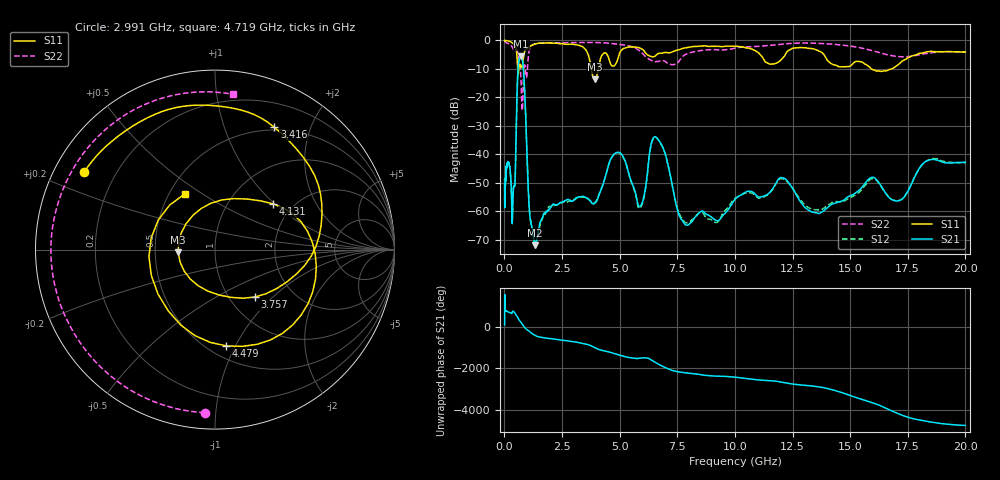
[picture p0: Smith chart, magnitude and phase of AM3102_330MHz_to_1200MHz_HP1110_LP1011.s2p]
! Date/Time: Tue, Sep 11, 2018 5:23 PM
! Network Analyzer: Agilent Technologies E8362B Rev: A.07.50.63
! Sweep from 0.010 to 20.000 GHz, 1601 Points, Sweep Type: LOG
! Power Supply: 4.949 V, 0.001 A
# Hz S DB R 50
!freq MagS11 AngS11 MagS21 AngS21 MagS12 AngS12 MagS22 AngS22
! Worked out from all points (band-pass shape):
!   1601 points, 10 MHz to 20 GHz, reference 50 ohm
!   highest |S21| = -5.65 dB at 726 MHz (marker M1); lowest = -72.0 dB at 1.34 GHz (marker M2)
!   |S21| within 3 dB of the highest: 603.5 MHz to 810.2 MHz (206.7 MHz wide, 29.2 % of centre)
!   lowest |S11| = -13.7 dB at 3.921 GHz (marker M3), VSWR 1.52, Z = 33 - j1.1 ohm
!   |S11| at or under -10 dB: 573.5 MHz to 626 MHz (52.43 MHz wide, 8.74 % of centre); 3.772 GHz to 4.081 GHz (308.9 MHz wide, 7.87 % of centre); 15.91 GHz to 16.81 GHz (895.3 MHz wide, 5.47 % of centre)
!   |S22| runs from -24.6 to -0.2 dB; largest |S21 - S12| = 0.0074
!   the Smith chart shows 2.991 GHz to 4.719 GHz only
!   S11 on the Smith chart (normalised r, x): 2.991 GHz: 0.09, +0.27; 3.416 GHz: 0.47, +1.49; 3.757 GHz: 1.30, -0.78; 4.131 GHz: 1.58, +0.97; 4.479 GHz: 0.61, -0.92; 4.719 GHz: 0.60, +0.43
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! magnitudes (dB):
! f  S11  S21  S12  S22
! 10 MHz  -0.1  -50.4  -48.5  -0.2
! 35.55 MHz  -0.1  -51.4  -51.4  -0.5
! 126.4 MHz  -0.2  -43.4  -43.1  -1.0
! 244.6 MHz  -0.5  -45.2  -45.2  -1.5
! 339.5 MHz  -1.0  -64.1  -63.3  -2.4
! 447.2 MHz  -1.8  -51.2  -51.6  -3.8
! 583.5 MHz  -11.4  -11.1  -11.1  -4.5
! 726 MHz  -9.4  -5.7  -5.7  -14.6
! 1.098 GHz  -2.2  -60.7  -60.7  -3.0
! 1.34 GHz  -1.3  -72.0  -71.7  -1.2
! 1.59 GHz  -1.0  -63.2  -63.7  -1.0
! 2.991 GHz  -1.4  -56.2  -55.9  -0.8
! 3.416 GHz  -2.4  -54.8  -55.0  -0.8
! 3.757 GHz  -9.3  -56.7  -56.5  -0.8
! 3.921 GHz  -13.7  -57.1  -57.0  -0.8
! 4.131 GHz  -7.7  -53.6  -53.6  -0.8
! 4.479 GHz  -5.4  -45.1  -44.9  -1.0
! 4.719 GHz  -9.0  -40.3  -40.4  -1.2
! 5.652 GHz  -2.4  -52.6  -53.1  -2.6
! 6.58 GHz  -5.3  -34.0  -34.1  -7.5
! 7.92 GHz  -2.5  -64.9  -64.1  -4.8
! 20 GHz  -4.1  -42.7  -43.1  -4.1
